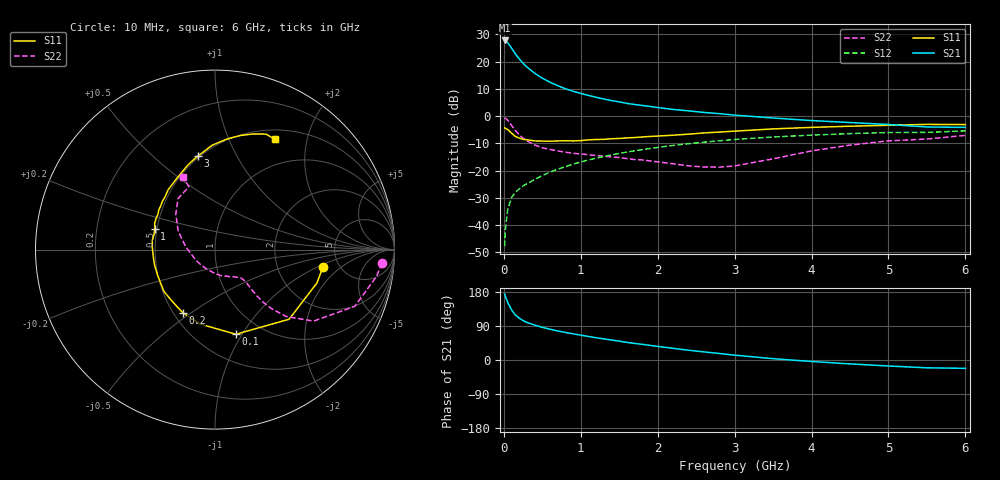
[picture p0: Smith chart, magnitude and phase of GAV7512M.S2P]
! Infineon Technologies  Discrete & RF Semiconductors
! BF775
! Si NPN RF Bipolar Junction Transistor in SOT23
! VCE = 0.75 V  IC = 12 mA
! Common Emitter S-Parameters:  May  1996
# GHz  S  MA  R  50
!  f  S11  S21  S12  S22
! GHz  MAG  ANG  MAG  ANG  MAG  ANG  MAG  ANG
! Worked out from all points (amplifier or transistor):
!   36 points, 10 MHz to 6 GHz, reference 50 ohm
!   highest |S21| = 27.8 dB at 10 MHz (marker M1)
!   |S21| within 3 dB of that: start of sweep to 104.4 MHz
!   unconditionally stable (mu >= 1): 349.5 MHz to end of sweep
!   at 250 MHz: K = 0.85, MSG = 22.5 dB, |S12| = -25.6 dB
!   at 1.4 GHz: K = 1.23, MAG = 7.1 dB, |S12| = -14.2 dB
!   at 6 GHz: K = 1.07, MAG = -1.0 dB, |S12| = -5.4 dB
!   S11 on the Smith chart (normalised r, x): 10 MHz: 3.73, -1.16; 100 MHz: 0.76, -0.94; 200 MHz: 0.56, -0.46; 1 GHz: 0.49, +0.13; 3 GHz: 0.49, +0.71; 6 GHz: 0.62, +1.49
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0.01  0.6092 -9.2  24.43 174.1  0.0041 85.5  0.9329 -4.6
0.02  0.5976 -18.1  24.18 167.8  0.0081 81.1  0.9124 -9.4
0.05  0.5667 -43.2  22.24 151.9  0.0193 71.5  0.8404 -22.1
0.1  0.4858 -76.1  17.67 132.3  0.0321 61.7  0.6781 -36.0
0.15  0.423 -101.0  13.83 118.7  0.0399 57.2  0.5446 -43.2
0.2  0.3947 -117.2  11.24 110.3  0.0462 56.6  0.4546 -46.3
0.25  0.3735 -130.1  9.312 104.0  0.0523 56.8  0.3941 -47.6
0.3  0.3677 -140.7  7.923 99.1  0.0573 57.7  0.3513 -47.8
0.4  0.3505 -156.0  6.118 92.1  0.0686 59.8  0.2954 -47.4
0.5  0.3477 -166.1  4.966 86.2  0.0809 60.8  0.2631 -46.7
0.6  0.3462 -174.8  4.184 81.2  0.0938 61.5  0.2442 -46.5
0.7  0.3494 178.1  3.621 76.7  0.106 61.9  0.2299 -46.8
0.8  0.353 171.7  3.18 72.6  0.1185 61.6  0.2174 -47.4
1  0.3551 161.0  2.604 65.6  0.144 60.7  0.2019 -49.6
1.1  0.3662 156.7  2.395 62.1  0.1565 60.0  0.1956 -51.8
1.6  0.398 137.4  1.712 46.5  0.2187 54.7  0.1659 -64.3
2.2  0.4462 119.4  1.324 30.8  0.2892 46.7  0.1333 -90.1
3  0.5292 100.5  1.042 12.8  0.3716 35.0  0.1216 -150.5
3.5  0.582 91.5  0.922 3.5  0.4133 27.6  0.1642 174.4
4.5  0.6521 77.3  0.761 -10.3  0.4773 13.6  0.2936 138.1
5.5  0.7038 66.1  0.631 -20.6  0.5017 0.1  0.3792 112.5
6  0.6986 61.6  0.621 -22.0  0.5359 -3.7  0.4419 114.0
